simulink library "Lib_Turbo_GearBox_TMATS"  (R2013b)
settings: Solver=ode45  StartTime=0.0  StopTime=10.0  RelTol=1e-3
undefined symbols (not defined in the file or in its folder): Eff_M, R_M

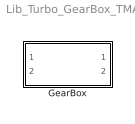
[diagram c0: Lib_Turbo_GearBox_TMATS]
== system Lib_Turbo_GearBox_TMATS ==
  GearBox : Subsystem

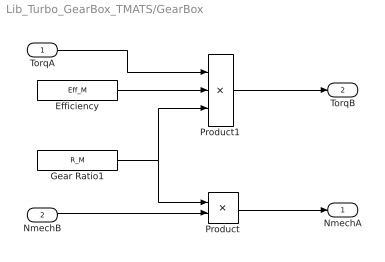
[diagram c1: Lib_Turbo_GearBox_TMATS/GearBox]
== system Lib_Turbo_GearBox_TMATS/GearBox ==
  TorqA : Inport
  NmechB : Inport  Port=2
  Efficiency : Constant  Value=Eff_M
  Gear Ratio1 : Constant  Value=R_M
  Product : Product
  Product1 : Product  Inputs=3
  NmechA : Outport
  TorqB : Outport  Port=2
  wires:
  Efficiency/1 -> Product1/2
  TorqA/1 -> Product1/1
  Gear Ratio1/1 -> Product1/3, Product/1
  NmechB/1 -> Product/2
  Product1/1 -> TorqB/1
  Product/1 -> NmechA/1
